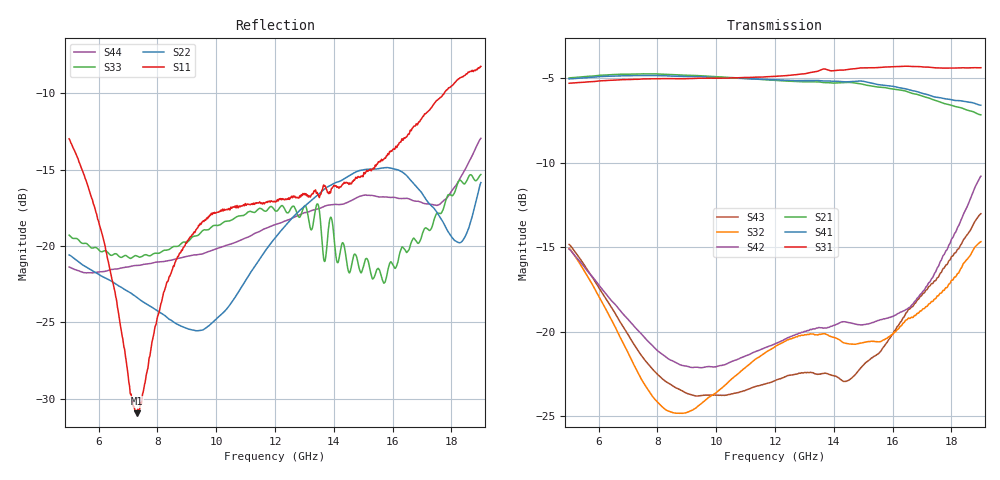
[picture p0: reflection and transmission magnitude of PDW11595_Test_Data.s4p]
!Keysight Technologies,N5227B,US57180409,A.15.40.08
!Date: Saturday, April 13, 2024 11:18:15
!Correction: S11(C  4-Port  )
!S12(C  4-Port  )
!S13(C  4-Port  )
!S14(C  4-Port  )
!S21(C  4-Port  )
!S22(C  4-Port  )
!S23(C  4-Port  )
!S24(C  4-Port  )
!S31(C  4-Port  )
!S32(C  4-Port  )
!S33(C  4-Port  )
!S34(C  4-Port  )
!S41(C  4-Port  )
!S42(C  4-Port  )
!S43(C  4-Port  )
!S44(C  4-Port  )
!S4P File: Measurements: <S11,S12,S13,S14>,
!<S21,S22,S23,S24>,
!<S31,S32,S33,S34>,
!<S41,S42,S43,S44>:
# Hz S  dB  R 50
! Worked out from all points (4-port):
!   3201 points, 5 GHz to 19 GHz, reference 50 ohm
!   strongest paths, dB at 5 GHz, 8.5 GHz, 12 GHz, 15.5 GHz, 19 GHz:
!     S31: -5.3, -5.0, -4.9, -4.4, -4.4
!     S41: -5.0, -4.9, -5.1, -5.4, -6.6
!     S21: -5.0, -4.8, -5.1, -5.5, -7.2
!     S42: -15.1, -21.7, -20.7, -19.3, -10.8
!     S32: -15.1, -24.8, -20.9, -20.6, -14.7
!     S43: -14.8, -23.2, -22.9, -21.3, -13.0
!   lowest |S11| = -31.0 dB at 7.301 GHz (marker M1), VSWR 1.06, Z = 50.1 - j2.84 ohm
!   |S11| at or under -10 dB: start of sweep to 17.75 GHz
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5e9  -12.99 60.4  -5.01 -118.3  -5.33 -120.9  -5.08 -118.6
     -4.99 -118.3  -20.59 -56.7  -15.06 -98.4  -15.12 172.7
     -5.30 -120.9  -15.06 -98.4  -19.29 94.0  -14.85 -96.1
     -5.05 -118.6  -15.11 172.6  -14.84 -96.1  -21.38 -68.7
7.30125e9  -30.95 -85.8  -4.76 -177.5  -5.07 -179.7  -4.85 -177.5
           -4.76 -177.5  -23.37 -146.3  -22.28 -109.7  -19.84 86.1
           -5.07 -179.8  -22.28 -109.8  -20.66 37.8  -21.00 -108.7
           -4.85 -177.5  -19.84 86.1  -21.00 -108.6  -21.28 -167.7
8.68375e9  -20.72 154.0  -4.80 146.1  -5.02 144.4  -4.87 146.5
           -4.80 146.1  -25.13 160.4  -24.80 -89.1  -21.87 22.4
           -5.03 144.3  -24.81 -89.2  -20.03 -3.6  -23.35 -99.1
           -4.88 146.5  -21.88 22.5  -23.35 -99.0  -20.82 146.3
1.0705e10  -17.37 66.0  -4.99 93.0  -4.97 92.2  -4.99 93.8
           -4.99 93.1  -23.17 61.7  -22.53 -73.7  -21.64 -68.5
           -4.98 92.1  -22.54 -73.9  -18.09 -46.2  -23.60 -87.3
           -5.01 93.9  -21.64 -68.5  -23.60 -87.2  -19.73 75.6
1.414812e10  -16.16 -116.2  -5.29 1.7  -4.55 1.1  -5.23 2.6
             -5.28 1.7  -15.80 -37.9  -20.44 -98.3  -19.54 157.0
             -4.53 0.8  -20.43 -98.5  -21.06 -86.4  -22.72 -91.2
             -5.19 2.4  -19.51 156.8  -22.70 -91.1  -17.30 -36.7
1.67775e10  -12.13 100.0  -5.92 -72.6  -4.38 -73.0  -5.80 -71.1
            -5.94 -72.9  -16.06 -104.9  -19.13 -99.5  -18.21 31.9
            -4.31 -73.4  -19.04 -99.6  -19.63 -41.9  -18.26 -86.0
            -5.77 -71.6  -18.16 31.7  -18.30 -86.2  -17.07 -132.6
1.9e10  -8.26 7.7  -7.04 -132.5  -4.34 -136.6  -6.52 -131.9
        -7.17 -132.3  -15.86 89.4  -14.76 -116.2  -10.85 -94.5
        -4.38 -136.1  -14.67 -115.9  -15.33 -39.9  -12.99 -109.6
        -6.60 -131.6  -10.80 -94.5  -13.02 -109.9  -12.96 90.6
